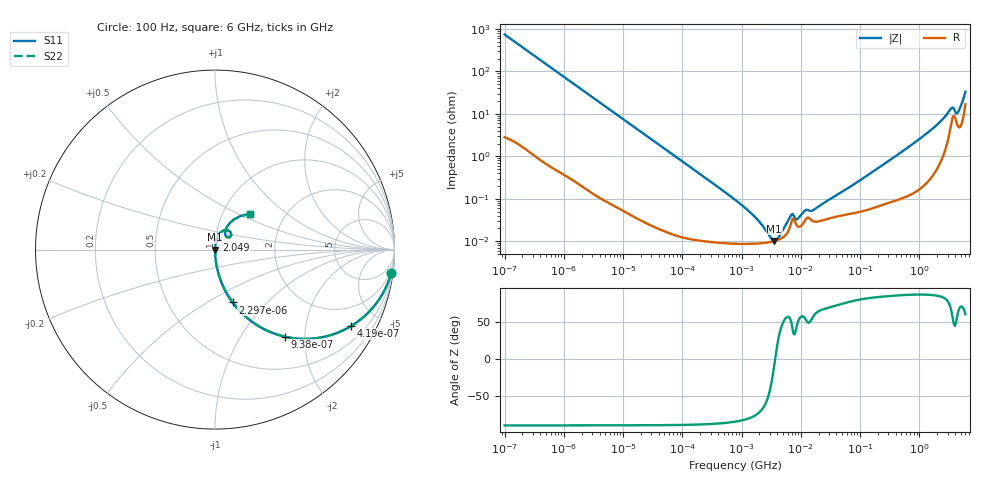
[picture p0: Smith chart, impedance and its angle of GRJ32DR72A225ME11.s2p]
!Murata Part Number: GRJ32DR72A225ME11
!These Parameters are Measured in Series Mode Connection
!Data Generated on Jun 19, 2026
!  o--ll--o
!Port1  Port2
!  o------o
!Operation Temp=25[degC], DC Bias Voltage=0[V]
!Freq. Start=100[Hz] Stop=6[GHz] 401[Steps]
# Hz S RI R 50
!Freq.(Hz) S11(Real) S11(Imag) S21(Real) S21(Imag) S12(Real) S12(Imag) S22(Real) S22(Imag)
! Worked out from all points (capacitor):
!   401 points, 100 Hz to 6 GHz, reference 50 ohm
!   read as one part in series: C = 2.13 uF near 109 Hz
!   lowest |Z| = 10.2 mohm at 3.55 MHz (marker M1)
!   series resonance near 3.691 MHz, so ESL is about 870 pH
!   S11 on the Smith chart (normalised r, x): 100 Hz: 1, -15; 419 Hz: 1.02, -3.57; 938 Hz: 1.01, -1.60; 2.297 kHz: 1.00, -0.65; 2.049 GHz: 1.01, +0.11; 6 GHz: 1.34, +0.58
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100  0.9818 -0.1318  0.0182 0.1318  0.0182 0.1318  0.9818 -0.1318
224  0.9165 -0.2745  0.0835 0.2745  0.0835 0.2745  0.9165 -0.2745
419  0.7601 -0.4248  0.2399 0.4248  0.2399 0.4248  0.7601 -0.4248
627  0.5873 -0.49  0.4127 0.49  0.4127 0.49  0.5873 -0.49
938  0.3901 -0.4853  0.6099 0.4853  0.6099 0.4853  0.3901 -0.4853
2008  0.1241 -0.3271  0.8759 0.3271  0.8759 0.3271  0.1241 -0.3271
2297  0.098 -0.2947  0.902 0.2947  0.902 0.2947  0.098 -0.2947
7695  0.0101 -0.097  0.9899 0.097  0.9899 0.097  0.0101 -0.097
40335  0.000548 -0.0188  0.9995 0.0188  0.9995 0.0188  0.000548 -0.0188
774597  8.82e-05 -0.000948  0.9999 0.000948  0.9999 0.000948  8.82e-05 -0.000948
1734173  8.79e-05 -0.000347  0.9999 0.000347  0.9999 0.000347  8.79e-05 -0.000347
3549919  0.000101 -1.67e-05  0.9999 1.67e-05  0.9999 1.67e-05  0.000101 -1.67e-05
4246196  0.000109 6.14e-05  0.9999 -6.14e-05  0.9999 -6.14e-05  0.000109 6.14e-05
6948629  0.000284 0.000316  0.9997 -0.000316  0.9997 -0.000316  0.000284 0.000316
8692127  0.000228 0.000238  0.9998 -0.000238  0.9998 -0.000238  0.000228 0.000238
1.189169e7  0.000317 0.000432  0.9997 -0.000432  0.9997 -0.000432  0.000317 0.000432
1.555665e7  0.000304 0.00043  0.9997 -0.00043  0.9997 -0.00043  0.000304 0.00043
3.124326e8  0.000873 0.00797  0.9991 -0.00797  0.9991 -0.00797  0.000873 0.00797
2.048624e9  0.00861 0.0565  0.9914 -0.0565  0.9914 -0.0565  0.00861 0.0565
3.352442e9  0.0563 0.1086  0.9437 -0.1086  0.9437 -0.1086  0.0563 0.1086
4.385646e9  0.0586 0.0785  0.9414 -0.0785  0.9414 -0.0785  0.0586 0.0785
6e9  0.1927 0.199  0.8073 -0.199  0.8073 -0.199  0.1927 0.199
